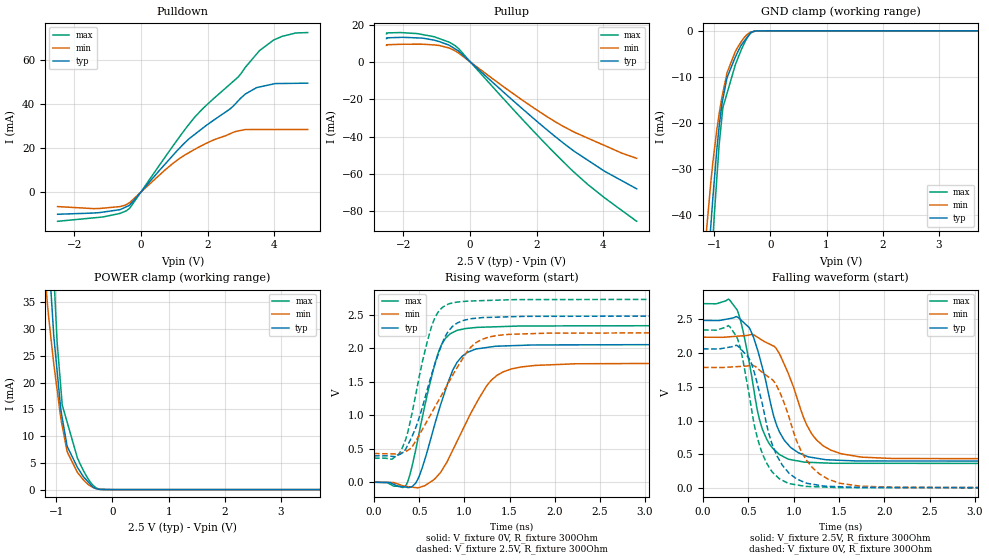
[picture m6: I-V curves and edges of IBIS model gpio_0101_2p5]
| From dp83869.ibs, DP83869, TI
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|   gpio_0101_2p5 Model
[Model]   gpio_0101_2p5
Model_type   I/O
Polarity   Non-Inverting
Enable   Active-Low
Vinl = 0.7
Vinh = 1.7
Vmeas = 1.25
Vref = 0
Cref = 2pF
Rref = 100000
|   typ   min   max
C_comp   1.246pF   1.092pF   1.323pF
| Where Nom  PVT is Nominal Process, 2.5V,  27C
|   Fast PVT is Strong Process,  2.75V, -40C
|   Slow PVT is Weak Process,   2.25V, 125C
[Voltage Range]   2.5   2.25   2.75
|Junction Temperature
[Temperature Range]   27   125   -40
[Pullup Reference]   2.5   2.25   2.75
[Pulldown Reference]   -0   -0   0
[Power Clamp Reference]   2.5   2.25   2.75
[GND Clamp Reference]   0   0   0
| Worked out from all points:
|   slope of the pulldown table from 0 to 0.375 V, typ, clamps not added: 56.2 ohm
|   slope of the pullup table from 0 to 0.375 V, typ, clamps not added: 60.9 ohm
|   GND clamp passes 1 mA (typ) near -0.39 V on its own axis
|   POWER clamp passes 1 mA (typ) near -0.39 V on its own axis
|   falling waveform, V_fixture 2.5V, R_fixture 300Ohm: 20-80 % time 254ps typ, 323ps min, 214ps max; typ from 2.49 V to 0.395 V
|   rising waveform, V_fixture 0V, R_fixture 300Ohm: 20-80 % time 286ps typ, 413ps min, 238ps max; typ from 0 V to 2.06 V
|   rising waveform, V_fixture 2.5V, R_fixture 300Ohm: 20-80 % time 293ps typ, 459ps min, 234ps max; typ from 0.395 V to 2.49 V
|   falling waveform, V_fixture 0V, R_fixture 300Ohm: 20-80 % time 264ps typ, 331ps min, 225ps max; typ from 2.06 V to 0 V
[Pulldown]
|   Voltage   I(typ)   I(min)   I(max)
-2.5V     -10.12mA   -6.627mA   -13.32mA
-1.258V   -9.396mA   -7.522mA   -11.53mA
-433.9mV  -6.689mA   -5.684mA   -8.526mA
-305.7mV  -5.387mA   -4.355mA   -6.712mA
1.303V    22.19mA    16.69mA    28.09mA
2.151V    32.34mA    23.5mA     42.08mA
2.906V    41.31mA    27.71mA    52.16mA
3.127V    44.51mA    28.39mA    56.64mA
3.556V    47.76mA    28.39mA    64.33mA
3.979V    49.15mA    28.4mA     69.11mA
4.636V    49.41mA    28.41mA    72.3mA
5V        49.49mA    28.41mA    72.49mA
[GND Clamp]
|   Voltage   I(typ)   I(min)   I(max)
-2.5V     -325.5mA   -278mA     -374.2mA
-1.151V   -58.23mA   -45.14mA   -72.46mA
-1.062V   -42.41mA   -32.96mA   -53.35mA
-1.027V   -36.66mA   -28.83mA   -45.97mA
-1.003V   -32.98mA   -26.33mA   -40.68mA
-915.3mV  -20.96mA   -18.2mA    -25.04mA
-847.2mV  -14.86mA   -13.48mA   -16.68mA
-770.2mV  -10.08mA   -9.023mA   -13.46mA
-624.7mV  -5.69mA    -4.486mA   -7.363mA
-460.9mV  -2.148mA   -1.394mA   -2.584mA
-358.7mV  -493.6uA   -330.5uA   -624.1uA
5V        0A         0A         0A
[Pullup]
|   Voltage   I(typ)   I(min)   I(max)
-2.5V     12.63mA    8.996mA    15.21mA
-2.084V   13.27mA    9.553mA    15.86mA
-1.378V   12.76mA    9.571mA    14.64mA
-917.2mV  11.02mA    8.909mA    12.61mA
-624.7mV  9.105mA    7.581mA    10.72mA
-457.2mV  7.247mA    6.173mA    9.007mA
-316.2mV  5.515mA    4.517mA    6.81mA
1.555V    -24.78mA   -20.21mA   -30.39mA
2.568V    -40.13mA   -32.13mA   -49.35mA
3.532V    -52.65mA   -40.8mA    -65.66mA
4.025V    -58.46mA   -44.67mA   -72.67mA
5V        -68mA      -51.65mA   -85.45mA
[POWER Clamp]
|   Voltage   I(typ)   I(min)   I(max)
-2.5V     383.1mA    300.3mA    465.8mA
-1.265V   71.44mA    49.26mA    97.29mA
-1.162V   48.95mA    35.07mA    69.59mA
-1.083V   35.06mA    27.13mA    48.54mA
-1.045V   28.71mA    23.46mA    40.28mA
-931.5mV  16.22mA    14.27mA    20.57mA
-895mV    13.42mA    11.91mA    15.83mA
-802.5mV  7.998mA    6.976mA    12.44mA
-624.4mV  4.167mA    3.23mA     5.922mA
-448.9mV  1.629mA    1.119mA    2.268mA
-321.9mV  342.6uA    265.3uA    574.8uA
5V        0A         0A         0A
[Ramp]
R_load = 300
|   typ   min   max
dV/dt_r   1.23683/2.85069e-10   1.07057/4.12229e-10   1.40538/2.37539e-10
dV/dt_f   1.25461/2.51847e-10   1.08432/3.20992e-10   1.42429/2.12303e-10
[Falling Waveform]
V_fixture = 2.5V
V_fixture_min = 2.25V
V_fixture_max = 2.75V
R_fixture = 300Ohm
C_fixture = 0F
|   Time   V(typ)   V(min)   V(max)
0s        2.486V     2.237V     2.734V
296.4ps   2.513V     2.243V     2.784V
403.5ps   2.511V     2.254V     2.536V
509.9ps   2.376V     2.269V     1.86V
658.1ps   1.77V      2.187V     861.5mV
806.4ps   951.8mV    2.071V     541.6mV
936.5ps   646.5mV    1.713V     429.5mV
1.2ns     452.2mV    802.5mV    377.5mV
1.528ns   408.4mV    505.8mV    365.1mV
5ns       394.8mV    429.5mV    360.6mV
[Rising Waveform]
V_fixture = 0V
V_fixture_min = 0V
V_fixture_max = 0V
R_fixture = 300Ohm
C_fixture = 0F
|   Time   V(typ)   V(min)   V(max)
0s        165.9uV    287.3uV    163.6uV
357.5ps   -73.33mV   -61.88mV   -36.66mV
488.5ps   55.31mV    -81.99mV   663.7mV
703.9ps   1.01V      97.37mV    1.907V
787.5ps   1.364V     257.8mV    2.144V
912.5ps   1.775V     593.2mV    2.264V
1.037ns   1.94V      936.9mV    2.298V
1.254ns   2.014V     1.452V     2.317V
1.532ns   2.04V      1.696V     2.329V
5ns       2.062V     1.785V     2.342V
[Rising Waveform]
V_fixture = 2.5V
V_fixture_min = 2.25V
V_fixture_max = 2.75V
R_fixture = 300Ohm
C_fixture = 0F
|   Time   V(typ)   V(min)   V(max)
0s        394.8mV    429.5mV    360.6mV
196ps     387.5mV    423.4mV    343.8mV
305.8ps   431.7mV    438.1mV    495.2mV
363.1ps   528.8mV    468.6mV    696.1mV
456ps     795.4mV    605mV      1.273V
639.5ps   1.618V     1.041V     2.339V
824.7ps   2.259V     1.487V     2.662V
1.077ns   2.442V     2.026V     2.707V
1.375ns   2.466V     2.193V     2.719V
5ns       2.486V     2.237V     2.734V
[Falling Waveform]
|Gnd
V_fixture = 0V
V_fixture_min = 0V
V_fixture_max = 0V
R_fixture = 300Ohm
C_fixture = 0F
|   Time   V(typ)   V(min)   V(max)
0s        2.063V     1.788V     2.343V
300.6ps   2.091V     1.793V     2.383V
409ps     2.073V     1.802V     2.088V
505.4ps   1.928V     1.813V     1.414V
672.6ps   1.131V     1.693V     453mV
758.9ps   661.8mV    1.613V     246.5mV
936.5ps   237.6mV    1.105V     70.03mV
1.145ns   68.88mV    406.1mV    21.29mV
1.508ns   16.7mV     69.28mV    4.726mV
5ns       163.1uV    282.9uV    162.7uV
